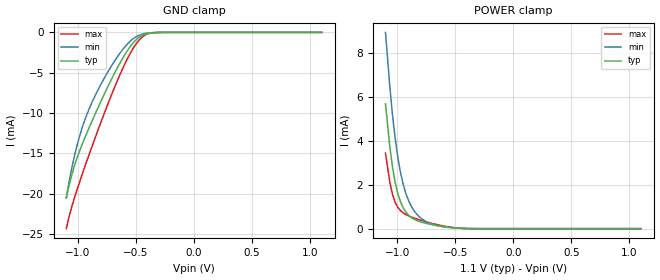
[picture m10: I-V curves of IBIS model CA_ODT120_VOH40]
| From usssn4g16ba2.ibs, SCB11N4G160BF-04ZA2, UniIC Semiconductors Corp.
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|   Model CA_ODT120_VOH40
[Model] CA_ODT120_VOH40
Model_type Input
Vinl =  0.130V
Vinh =  0.310V
C_comp   0.710pF   0.700pF   0.720pF
[Model Spec]
Vinh   0.310V   0.302V   0.324V
Vinl   0.130V   0.122V   0.144V
[Add Submodel]
|  Submodel_name   Mode
ODT120_VOH40_CACLK   Non-Driving
[Temperature Range]   25.000   0.105k   -40.000
[Voltage Range]   1.100V   1.060V   1.170V
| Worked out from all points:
|   GND clamp passes 1 mA (typ) near -0.51 V on its own axis
|   POWER clamp passes 1 mA (typ) near -0.95 V on its own axis
[GND_clamp]
|Voltage   I(typ)   I(min)   I(max)
-1.1V     -20.5mA    -20.51mA   -24.31mA
-1.054V   -17.69mA   -16.89mA   -21.65mA
-1.008V   -15.57mA   -14.02mA   -19.49mA
-939mV    -13.01mA   -10.79mA   -16.57mA
-870mV    -10.71mA   -8.379mA   -13.79mA
-732mV    -6.413mA   -4.649mA   -8.508mA
-594mV    -2.707mA   -1.765mA   -3.85mA
-502mV    -951.2uA   -567uA     -1.477mA
-433mV    -266.6uA   -164.4uA   -430.6uA
-387mV    -88.17uA   -61.66uA   -135.3uA
-295mV    -6.313uA   -6.787uA   -6.983uA
1.1V      0A         0A         0A
[POWER_clamp]
|Voltage   I(typ)   I(min)   I(max)
-1.1V     5.671mA    8.923mA    3.433mA
-1.062V   3.7mA      6.421mA    2.09mA
-1.039V   2.777mA    5.138mA    1.545mA
-1.016V   2.084mA    4.076mA    1.192mA
-970mV    1.209mA    2.536mA    818.5uA
-947mV    943.5uA    2.003mA    716.7uA
-901mV    610.1uA    1.27mA     581.3uA
-855mV    430.7uA    824uA      484.6uA
-786mV    289.9uA    439.4uA    366uA
-671mV    155.9uA    155.9uA    203.6uA
-441mV    13.2uA     12.79uA    15.03uA
1.1V      0A         0A         0A
